//FC654.AWL
// ***************************************************************************

FUNCTION "FC_SR_ASTA" : VOID
TITLE = Querkopplung ASTA-Aufträge abarbeiten

AUTHOR: 	SIEMENS
FAMILY: 	SISTARS7
NAME:      XCASTA
VERSION: 	4.02

//KNOW_HOW_PROTECT

// Datum	Name			Aktion
// ---------------------------------------------------------------------------
// 25.06.99 Mahler		Neu

VAR_INPUT
     iFKT		:INT;			//1=Senden 2=Empfang
END_VAR


VAR_TEMP
	//Offset LW0!!!
	u			: "XC_ASTA_UDT";

	iRecord		: INT;
	i			: INT;
	dwAR1			: DWORD;
	wDB_NUMBER		: WORD;
     	iRetVal		: INT;
	wDB_LENGTH		: WORD;
	dDestByte		: DINT;
	boWRITE_PROT	: BOOL;
END_VAR

BEGIN


NETWORK
TITLE = Prüfen ob XC_ASTA_RCV vorhanden
// ===========================================================================

	L #iFKT;			//Funktion 72 = Teilanlagenstart ausführen von S7
	L 72;
	==I;
	spb anfS;

	L #iFKT;			//Funktion 52 = Teilanlagenstart ausführen von S5
	L 52;
	==I;
	spb anfS;
	beb;

anfS:	L	988;
	T	#wDB_NUMBER;

	CALL "TEST_DB"
	(
           DB_NUMBER		:= #wDB_NUMBER,
           RET_VAL      	:= #iRetVal,
		DB_LENGTH		:= #wDB_LENGTH,
		WRITE_PROT		:= #boWRITE_PROT
	);

	L     #iRetVal;
	L     0;
	<>I   ; 					//Fehler: DB nicht vorhanden
	BEB;


NETWORK
TITLE = XC_ASTA abarbeiten
// ===========================================================================

RUN:	L	"XC_RASTA_SR".iOffset;
	SLW	3;
	LAR1;

	L	1;
LOOP:	T	#iRecord;
	L	"XC_RASTA_SR".iAct;
	>I;
	SPB	EXIT;

	//Datensatz in Lokaldaten kopieren
	L	DBD	[AR1, P#0.0];
	T	LD	0;

	L	#u.bDestPCU;
	L	0;
	==I;
	SPB	NEXT;					//Datensatz abgearbeitet

	L	#u.bDestPCU;
	L	254;
	>=I;
	SPB	NEXT;					//Datensatz fehlerhaft

	L	DBD	[AR1, P#4.0];
	T	LD	4;
	L	DBD	[AR1, P#8.0];
	T	LD	8;

	TAR1	#dwAR1;				//AR1 retten

	L	#u.bDestSEQ;
	T	#i;

	CALL	"ATTRIB_PTR_FC"
	(
  		iDB 			:= 725,
		iRecord 		:= i,
  		iRelByteOffset 	:= 0,
  		iRetVal 		:= #iRetVal
	);

	L	#u.bSrcASTA;
	+	-1;
	L	"ASTA".iLen;
	*I;
	L	"ASTA".iOffset;
	+I;
	+	4;					//bRemoteErr
	T	#dDestByte;

	L	#u.bSrcPCU;
	T	#i;

	L	#iRetVal;
	L	0;
	<>I;
	SPB	ERR;

	AUF	"TA";

	UN	DBX	[AR1, P#7.6];		//TA: boDB Dauerbedingung nicht erfüllt
	SPB	SERR;

	U	DBX	[AR1, P#7.7];		//TA: boHAND Handbetrieb
	SPB	SERR;

	L	DBW	[AR1, P#10.0];		//TA: byNewStep, byStep
	L	0;
	<>I;
	SPB	SERR;					//Teilanlage läuft

	//Alles claro, TA kann gestartet werden
	L	LD	4;				//bYear, bRecipeType, iRecipe
	T	DBD	[AR1, P#14.0];		//TA: s.o.

	L	0;
	L	LD	8;				//iOrder, iBatch
	==D;
	SPB	NSTP;					//Auftr.nr/Chargennr. in Ziel-TA nicht verändern!
	T	DBD	[AR1, P#18.0];		//TA: s.o.



NSTP: L   iFKT;
	L 52;
	==I;
      spb STAR;

	CALL	"FC_SR_JOB_USER"              //Fehler in Asta zuruecksenden nur wenn S7
	(
		iMode			:= 1,
		iJob			:= 0,				//SystemAuftrag 1 ... 32
		iPCU			:= #i,
		iType			:= 50,			//Sende
		boEnable		:= TRUE,
		boTmpJob		:= TRUE,
		iSrc_DType		:= 2,				//BYTE
		iSrc_AREA		:= 132,			//DB
		iSrc_DB		:= 984,
		dSrcByte		:= L#22,			//"Positive Quittung
		iSrcBit		:= 0,
		iSrc_Num		:= 2,
		iDest_DType		:= 2,				//BYTE
		iDest_AREA		:= 132,			//DB
		iDest_DB		:= 742,			//"ASTA"
		dDestByte		:= #dDestByte,
		iDestBit		:= 0,
		iTime			:= 0,
		iActTime		:= 0,
		boTms			:= 0,
		boTsec		:= 0,
		boTmin		:= 0,
		iRetVal		:= #iRetVal
	);

	L	#iRetVal;		//<=0: Fehler; >0: Belegter XC_JOB-Datensatz
	L	0;
	<=I;
	L	253;			//unquittierter Startfehler
	SPB	DPCU;			//später erneut versuchen!!


STAR:	L	1;
	T	DBB	[AR1, P#10.0];		//TA: byNewStep := 1

	L	0;
	SPA	DPCU;

ERR:	L	255;					//Daten als fehlerhaft markieren
	SPA	DPCU;

	//Startfehler zurückmelden
SERR: L   iFKT;
	L 52;
	==I;
      spb FERT;

	CALL	"FC_SR_JOB_USER"              //Fehler in Asta zuruecksenden nur wenn S7
	(
		iMode			:= 1,
		iJob			:= 0,				//SystemAuftrag 1 ... 32
		iPCU			:= #i,
		iType			:= 50,			//Sende
		boEnable		:= TRUE,
		boTmpJob		:= TRUE,
		iSrc_DType		:= 2,				//BYTE
		iSrc_AREA		:= 132,			//DB
		iSrc_DB		:= 984,
		dSrcByte		:= L#24,			//"Negative Quittung
		iSrcBit		:= 0,
		iSrc_Num		:= 2,
		iDest_DType		:= 2,				//BYTE
		iDest_AREA		:= 132,			//DB
		iDest_DB		:= 742,			//"ASTA"
		dDestByte		:= #dDestByte,
		iDestBit		:= 0,
		iTime			:= 0,
		iActTime		:= 0,
		boTms			:= 0,
		boTsec		:= 0,
		boTmin		:= 0,
		iRetVal		:= #iRetVal
	);

	L	#iRetVal;		//<=0: Fehler; >0: Belegter XC_JOB-Datensatz
	L	0;
	<=I;
	L	253;			//unquittierter Startfehler
	SPB	DPCU;			//später erneut versuchen!!

FERT:	L	254;			//quittierter Startfehler: Datensatz abgearbeitet
DPCU:	T	#u.bDestPCU;

	LAR1	#dwAR1;				//AR1 zurück ----

	AUF	"XC_RASTA_SR";

	L	#u.bDestPCU;
	T	DBB	[AR1, P#1.0];

NEXT:	L	"XC_RASTA_SR".iLen;
	SLW	3;
	+AR1;

	L	#iRecord;
	+	1;
	SPA	LOOP;

EXIT:	BEA;

END_FUNCTION

